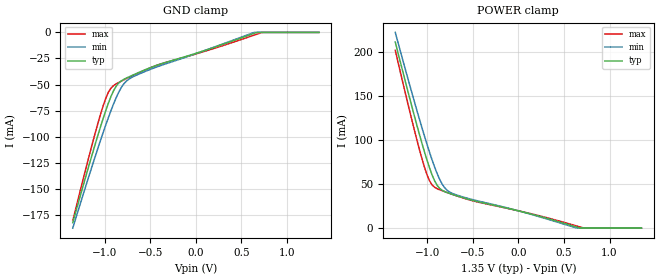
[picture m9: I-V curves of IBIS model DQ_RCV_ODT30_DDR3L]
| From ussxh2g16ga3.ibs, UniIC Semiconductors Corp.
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|   Model DQ_RCV_ODT30_DDR3L
[Model] DQ_RCV_ODT30_DDR3L
Model_type Input
Vinl =  0.540V
Vinh =  0.810V
C_comp   0.966pF   0.965pF   0.967pF
[Model Spec]
Vinh   0.810V   0.776V   0.860V
Vinl   0.540V   0.506V   0.590V
[Temperature Range]   25.000   95.000   -40.000
[Voltage Range]   1.350V   1.283V   1.450V
[GND_clamp]
|Voltage   I(typ)   I(min)   I(max)
-1.35V    -182.5mA   -187.7mA   -180.5mA
-1.126V   -113.8mA   -125mA     -103.7mA
-1.042V   -89.53mA   -102.6mA   -77.55mA
-986mV    -74.5mA    -88.3mA    -62.79mA
-930mV    -61.28mA   -74.79mA   -53.33mA
-874mV    -51.6mA    -62.66mA   -49.38mA
-818mV    -46.56mA   -52.94mA   -46.81mA
-762mV    -43.83mA   -46.72mA   -44.39mA
-398mV    -30.63mA   -32.19mA   -30.71mA
638mV     -1.014mA   -110.4uA   -2.669mA
750mV     0A         0A         0A
1.35V     0A         0A         0A
[POWER_clamp]
|Voltage   I(typ)   I(min)   I(max)
-1.35V    210.9mA    221.8mA    201.5mA
-1.142V   127.8mA    144mA      111.8mA
-1.058V   96.41mA    114mA      78.98mA
-1.002V   77.05mA    95.03mA    60.56mA
-946mV    60.26mA    77.29mA    48.93mA
-890mV    48.39mA    61.66mA    44.66mA
-834mV    42.78mA    49.66mA    42.35mA
-778mV    40.18mA    42.64mA    40.25mA
-610mV    34.54mA    35.38mA    34.32mA
650mV     900.4uA    0A         2.158mA
734mV     0A         0A         0A
1.35V     0A         0A         0A
